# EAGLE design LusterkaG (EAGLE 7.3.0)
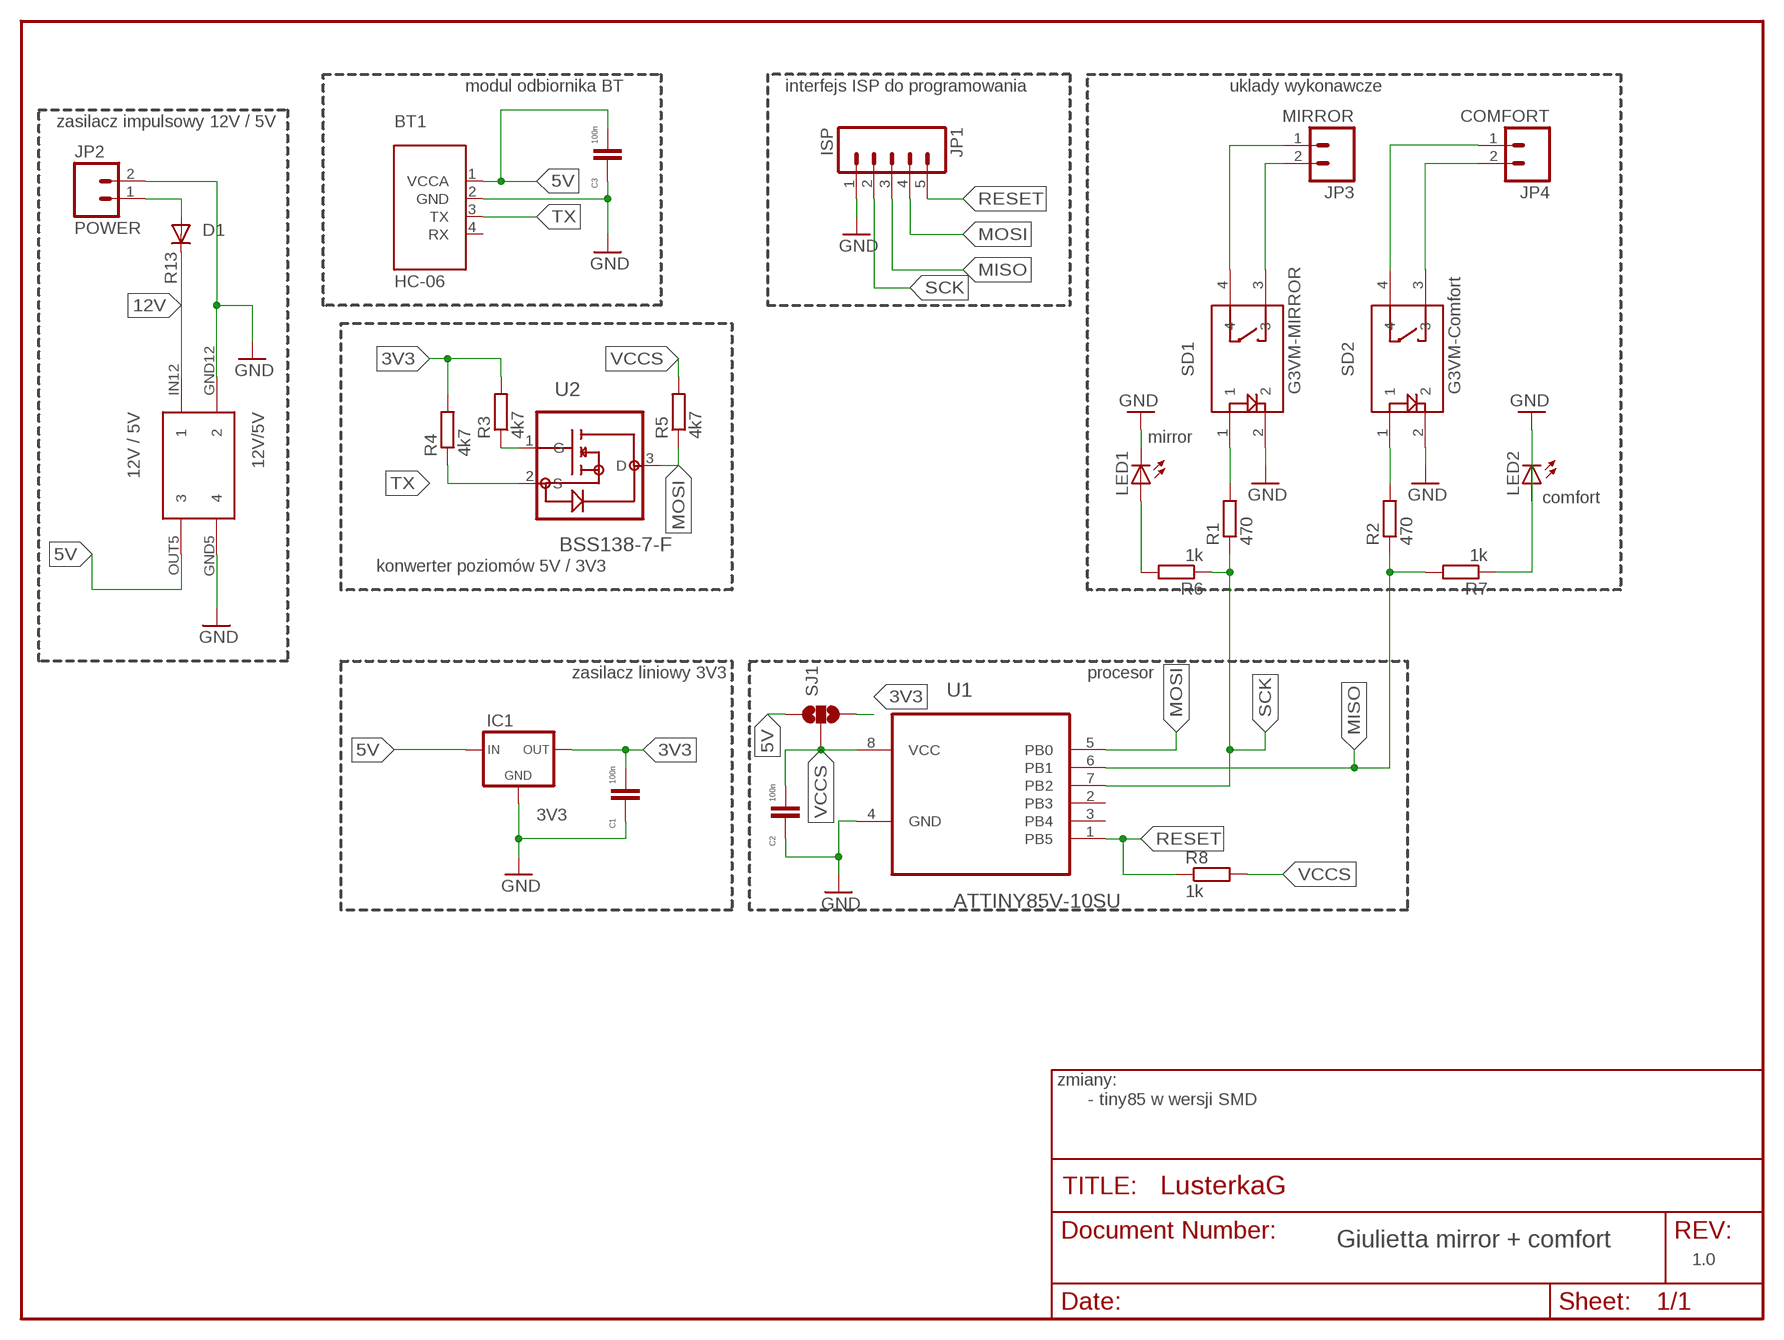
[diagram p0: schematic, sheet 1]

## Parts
12V/5V  12V / 5V  SWITCHING-POWER12V  [SWITCHING-POWER12V]
BT1  HC-06  HC-06-ADAPTER  [HC-06-ADAPETR-HORIZONTAL-V1]
C1  100n  C-EUC0805  [C0805]
C2  100n  C-EUC0805  [C0805]
C3  100n  C-EUC0805  [C0805]
D1  R13  ES2D  [SMB]
IC1  3V3  LM1117TO252  [TO252]
JP1  ISP  M05PTH  [1X05]
JP2  POWER  M02PTH  [1X02]
JP3  MIRROR  M02PTH  [1X02]
JP4  COMFORT  M02PTH  [1X02]
LED1  mirror  LEDCHIP-LED0603  [CHIP-LED0603]
LED2  comfort  LEDCHIP-LED0603  [CHIP-LED0603]
R1  470  R-EU_M0805  [M0805]
R2  470  R-EU_M0805  [M0805]
R3  4k7  R-EU_M0805  [M0805]
R4  4k7  R-EU_M0805  [M0805]
R5  4k7  R-EU_M0805  [M0805]
R6  1k  R-EU_M0805  [M0805]
R7  1k  R-EU_M0805  [M0805]
R8  1k  R-EU_M0805  [M0805]
SD1  G3VM-MIRROR  G3VM-SOLIDRELAY  [G3VM-SOLIDRELAY]
SD2  G3VM-Comfort  G3VM-SOLIDRELAY  [G3VM-SOLIDRELAY]
SJ1  SOLDERJUMPER_2WAYS  [SJ_3]
U1  ATTINY85V-10SU  [SOIC127P798X216-8N]
U2  BSS138-7-F  [SOT95P240X110-3N]

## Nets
3V3: C1.1 IC1.3(OUT) R3.2 R4.2 SJ1.3
5V: 12V/5V.OUT5 BT1.1(VCCA) C3.1 IC1.2(IN) SJ1.1
12V: D1.A JP2.1
GND: 12V/5V.GND5 12V/5V.GND12 BT1.2(GND) C1.2 C2.2 C3.2 IC1.1(GND) JP1.1 JP2.2 LED1.C LED2.A SD1.2 SD2.2 U1.4(GND)
MISO: JP1.3 R2.1 R7.2 U1.6(PB1)
MOSI: JP1.4 R5.1 U1.5(PB0) U2.3(D)
N$1: R1.2 SD1.1
N$2: R2.2 SD2.1
N$3: JP3.1 SD1.4
N$4: JP3.2 SD1.3
N$5: JP4.1 SD2.4
N$6: JP4.2 SD2.3
N$7: R3.1 U2.1(G)
N$8: LED1.A R6.2
N$9: LED2.C R7.1
N$10: 12V/5V.IN12 D1.C
RESET: JP1.5 R8.1 U1.1(PB5)
SCK: JP1.2 R1.1 R6.1 U1.7(PB2)
TX: BT1.3(TX) R4.1 U2.2(S)
VCCS: C2.1 R5.2 R8.2 SJ1.2 U1.8(VCC)
Unconnected: BT1.4(RX) U1.2(PB3) U1.3(PB4)

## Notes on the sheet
- modul odbiornika BT | interfejs ISP do programowania | uklady wykonawcze
- zasilacz impulsowy 12V / 5V
- konwerter poziomów 5V / 3V3
- zasilacz liniowy 3V3 | procesor
- zmiany:
- - tiny85 w wersji SMD
- Giulietta mirror + comfort
- 1.0

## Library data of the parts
12V/5V = switching_power_12V:SWITCHING-POWER12V: switching power from 12 V to +5V
BT1 = HC-05:HC-06-ADAPTER: HC06 4 pin horizontal 14x 100mil - 6x 100 mil
C1-C3 = lcd_C65-lbr:C-EU: CAPACITOR, European symbol
D1 = lcd_C65-lbr:ES2D: DIODE
IC1 = lcd_C65-lbr:LM1117
JP1 = SparkFun-Connectors:M05: Header 5 Standard 5-pin 0.1" header. Use with straight break away headers (SKU : PRT-00116), right angle break away headers (PRT-00553), swiss pins (PRT-00743), machine pins (PRT-00117), and female headers (PRT-00115). Molex polarized connector foot print use with SKU : PRT-08230 with associated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
JP2-JP4 = SparkFun-Connectors:M02: Standard 2-pin 0.1" header. Use with
LED1 LED2 = lcd_C65-lbr:LED: LED
R1-R8 = resistor:R-EU_: RESISTOR, European symbol
SD1 SD2 = G3VM-21GR1:G3VM-SOLIDRELAY: G3VM-21GR by Omron, 250 mA / 20 V
SJ1 = SparkFun-Passives:SOLDERJUMPER_2WAY: Solder Jumper 2 way solder jumper
U1 = Tiny85:ATTINY85V-10SU: 8-bit Microcontroller with In-System Programmable Flash; MPN: ATTINY85V-10SU; OC_FARNELL: 1455166; OC_NEWARK: 58M3799; PACKAGE: SOIC-8; SUPPLIER: Atmel
U2 = BSS138:BSS138-7-F: ENHANCEMENT MODE MOSFET; MPN: BSS138-7-F; OC_FARNELL: 1843693; OC_NEWARK: 12T1442; PACKAGE: SOT-23-3; SUPPLIER: DIODES INC.

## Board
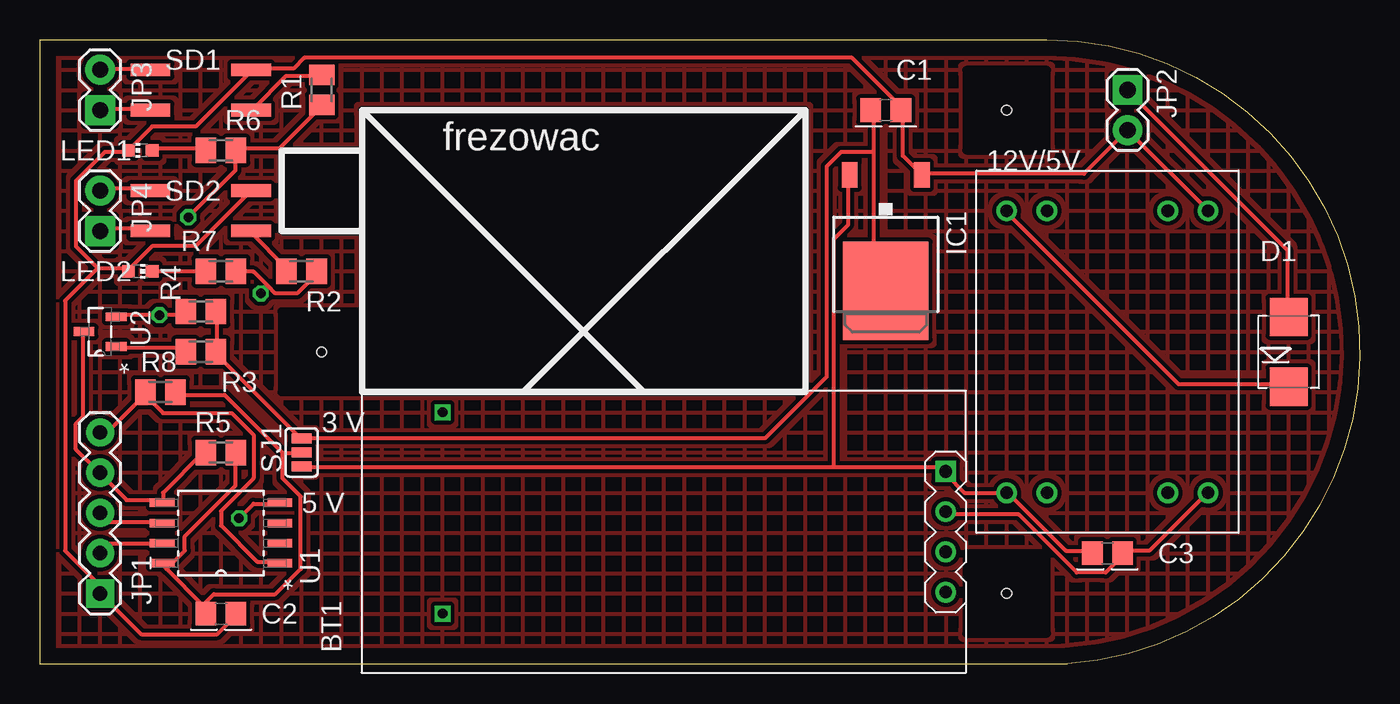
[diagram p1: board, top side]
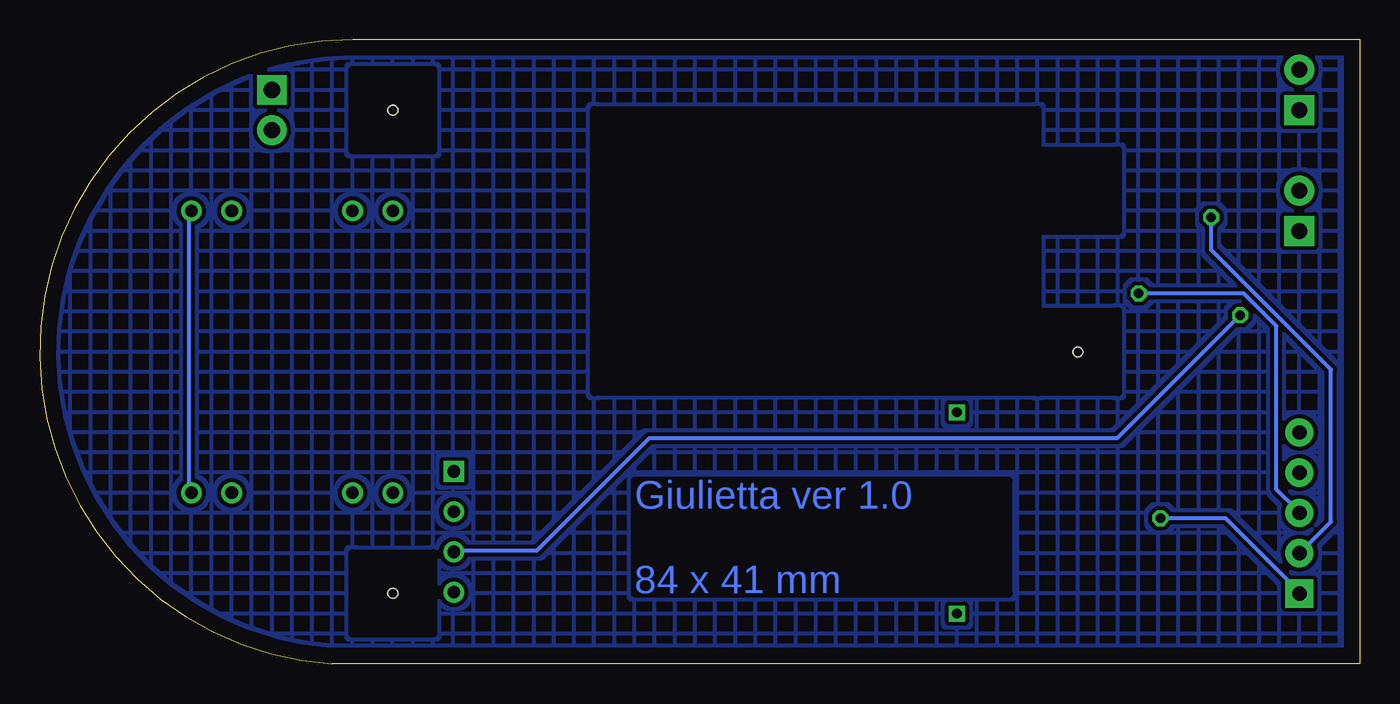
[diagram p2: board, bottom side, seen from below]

Size 83.22 x 39.37 mm. Coordinates in mm from the lower left corner, seen from the top.
Outline: 0,39.37 0,0 64.77,0 arc176 63.5,39.37 0,39.37
Copper layers (1*16): Top 0.035mm / dielectric 1.5mm / Bottom 0.035mm
Design rules "default *": minimum track width 10mil, minimum drill 0.6mm, track to track 8mil, track to pad 0.3mm, pad to pad 0.3mm, via to via 0.5mm, smd to smd 8mil, copper to edge 40mil, drill to drill 8mil, minimum pad ring 10mil, minimum via ring 8mil, stop-mask expansion 4mil, vias tented up to drill 0mil, thermal gap 10mil
Holes 0.6 mm at 60.96,34.93 60.96,4.45 17.78,19.68
tRestrict: area 20.3,17.1 to 48.3,34.9; area 15.2,27.3 to 20.3,32.4; area 15.2,17.1 to 20.3,22.2; area 58.4,32.4 to 63.5,37.5; area 58.4,1.9 to 63.5,7
bRestrict: area 20.3,17.1 to 48.3,34.9; area 15.2,27.3 to 20.3,32.4; area 15.2,17.1 to 20.3,22.2; area 58.4,32.4 to 63.5,37.5; area 58.4,1.9 to 63.5,7

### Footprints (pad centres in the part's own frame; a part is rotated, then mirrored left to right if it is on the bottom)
SWITCHING-POWER12V = drill 0.8: GND5 6.35,-8.89; GND5A 3.81,-8.89; GND12 6.35,8.89; GND12A 3.81,8.89; IN12 -6.35,8.89; IN12A -3.81,8.89; OUT5 -6.35,-8.89; OUT5A -3.81,-8.89
HC-06-ADAPETR-HORIZONTAL-V1 = drill 0.8 square: 1 5.08,0 | drill 0.8: 2 2.54,0; 3 0,0; 4 -2.54,0
C0805 = smd 1.3 x 1.5: 1 -0.95,0; 2 0.95,0
SMB = smd 2.4 x 2.4: A 2.2,0; C -2.2,0
TO252 = smd 1 x 1.6: 1 -2.28,-6.07; 2 2.28,-6.07 | smd 5.4 x 6.2: 3 0,1.23
1X05 = drill 0.9 pad 1.778 square: 1 0,0 | drill 0.9 pad 1.778: 2 2.54,0; 3 5.08,0; 4 7.62,0; 5 10.16,0
1X02 = drill 1.016 pad 1.88 square: 1 0,0 | drill 1.016 pad 1.88: 2 2.54,0
CHIP-LED0603 = smd 0.8 x 0.8: A 0,-0.75; C 0,0.75
M0805 = smd 1.3 x 1.6: 1 -0.95,0; 2 0.95,0
G3VM-SOLIDRELAY = smd 0.8 x 2.5: 1 -1.27,-3.175; 2 1.27,-3.175; 3 1.27,3.175; 4 -1.27,3.175
SJ_3 = smd 0.635 x 1.27: 1 -0.889,0; 2 0,0; 3 0.889,0
SOIC127P798X216-8N = smd 1.549 x 0.533: 1 -3.708,1.905; 2 -3.708,0.635; 3 -3.708,-0.635; 4 -3.708,-1.905; 5 3.708,-1.905; 6 3.708,-0.635; 7 3.708,0.635; 8 3.708,1.905
SOT95P240X110-3N = smd 1.321 x 0.559: 1 -1.016,0.94; 2 -1.016,-0.94; 3 1.016,0

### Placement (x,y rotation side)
12V/5V  67.31,19.68 0 top
BT1  57.12,7.07 90 top
C1  53.34,34.93 0 top
C2  11.43,3.17 0 top
C3  67.31,6.99 0 top
D1  78.74,19.68 90 top
IC1  53.34,24.76 180 top
JP1  3.81,4.45 90 top
JP2  68.58,36.2 270 top
JP3  3.81,34.93 90 top
JP4  3.81,27.3 90 top
LED1  6.35,32.39 90 top
LED2  6.35,24.76 270 top
R1  17.78,36.2 90 top
R2  16.51,24.76 180 top
R3  10.16,19.68 0 top
R4  10.16,22.22 0 top
R5  11.43,13.34 0 top
R6  11.43,32.39 180 top
R7  11.43,24.76 0 top
R8  7.62,17.14 0 top
SD1  10.16,36.2 90 top
SD2  10.16,28.57 90 top
SJ1  16.51,13.34 90 top
U1  11.43,8.26 180 top
U2  3.81,20.95 180 top

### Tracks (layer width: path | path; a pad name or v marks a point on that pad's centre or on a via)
3V3
  Top 0.254: R4.2 11.2,22.22 11.2,19.71 R3.2 11.2,19.48 16.46,14.22 SJ1.3 45.72,14.22 49.61,18.11 49.61,31.37 50.52,32.28 52.58,32.28 | 52.58,32.28 52.58,24.28 53.26,23.6 IC1.3 | 52.58,32.28 52.58,34.8 C1.1
5V
  Top 0.254: C3.1 66.29,7.14 64.69,7.14 61.04,10.79 12V/5V.OUT5 58.29,10.79 57.15,11.94 BT1.1 56.92,12.17 56.69,12.39 50.06,12.39 | 50.06,12.39 16.69,12.39 SJ1.1 | 50.06,12.39 50.06,26.8 50.98,27.71 50.98,30.68 IC1.2
12V
  Top 0.254: D1.A 78.64,22 78.64,26.11 68.58,36.17 JP2.1
GND  (via drill 0.6)
  Top 0.254: C2.2 12.34,3.02 11.2,1.88 6.4,1.88 3.89,4.39 JP1.1 3.66,4.62 3.66,5.08 1.6,7.14 1.6,22.91 3.66,24.97 | v12.57,9.2 13.49,10.11 15.09,10.11 U1.4 | SD2.2 9.83,26.34 7.09,26.34 5.71,24.97 LED2.A 5.49,24.97 3.66,24.97 | 3.66,24.97 2.29,26.34 2.29,30.45 4.12,32.28 5.49,32.28 LED1.C 5.71,32.51 7.09,33.88 9.83,33.88 13.26,37.31 SD1.2 13.49,37.54 16,37.54 16.69,38.23 51.21,38.23 54.41,35.03 C1.2 54.41,34.8 54.41,32.05 55.55,30.91 IC1.1 55.78,30.91 65.84,30.91 JP2.2 12V/5V.GND12 | 12V/5V.GND5 73.61,10.79 69.95,7.14 68.35,7.14 C3.2 68.35,6.91 67.21,5.77 65.38,5.77 61.72,9.42 57.15,9.42 BT1.2
  Bottom 0.254: v12.57,9.2 8.46,9.2 3.89,4.62 JP1.1 | 12V/5V.GND5 73.84,10.79 73.84,28.4 12V/5V.GND12
MISO  (via drill 0.6)
  Top 0.254: 14.4,23.82 14.86,23.37 16.23,23.37 17.6,24.74 R2.1 | 14.4,23.82 13.49,24.74 12.57,24.74 R7.2 | U1.6 7.54,8.97 4.34,8.97 3.89,9.42 JP1.3 | v13.95,23.37 14.4,23.82
  Bottom 0.254: v13.95,23.37 7.32,23.37 5.26,21.31 5.26,11.02 3.89,9.65 JP1.3
MOSI
  Top 0.254: R5.1 10.29,13.31 7.77,10.79 7.77,10.34 U1.5 7.54,10.34 5.49,10.34 3.89,11.94 JP1.4 3.66,12.17 2.29,13.54 2.29,15.14 2.74,15.6 2.74,20.85 U2.3
N$1
  Top 0.254: R1.2 17.6,37.08 15.54,37.08 13.49,35.03 SD1.1
N$2
  Top 0.254: R2.2 15.54,24.97 13.26,27.25 SD2.1
N$3
  Top 0.254: SD1.4 6.86,35.03 3.89,35.03 JP3.1
N$4
  Top 0.254: SD1.3 6.86,37.54 3.89,37.54 JP3.2
N$5
  Top 0.254: SD2.4 6.86,27.48 3.89,27.48 JP4.1
N$6
  Top 0.254: SD2.3 6.86,30 3.89,30 JP4.2
N$7
  Top 0.254: U2.1 5.03,19.94 8.91,19.94 9.14,19.71 R3.1
N$8
  Top 0.254: LED1.A 7.32,32.51 10.29,32.51 R6.2
N$9
  Top 0.254: LED2.C 7.32,24.74 10.29,24.74 R7.1
N$10
  Top 0.254: D1.C 78.64,17.65 71.78,17.65 61.04,28.4 12V/5V.IN12
N$11  (via drill 0.6)
  other vias: 25.4,15.88
N$12  (via drill 0.6)
  other vias: 25.4,3.17
N$13
  pour Top (isolate 0.254, hatched): 0,40.01 63.5,40.01 arc-90 83.82,19.68 arc-82 66.04,-0.64 0,-0.64
N$14
  pour Bottom (isolate 0.254, hatched): 0,40.01 63.5,40.01 arc-90 83.82,19.68 arc-82 66.04,-0.64 0,-0.64
RESET
  Top 0.254: 6.63,16.97 7.77,15.82 12.12,15.82 13.49,14.45 13.49,11.71 11.43,9.65 11.43,8.74 13.72,6.45 15.09,6.45 U1.1 | 6.63,16.97 4.34,14.68 3.89,14.68 JP1.5 | 6.63,16.97 R8.1
SCK  (via drill 0.6)
  Top 0.254: R1.1 17.6,35.03 15.09,32.51 12.57,32.51 R6.1 12.34,32.28 12.34,31.14 v9.37,28.17 | U1.7 7.54,7.6 4.34,7.6 3.89,7.14 JP1.2
  Bottom 0.254: v9.37,28.17 9.37,26.11 1.83,18.57 1.83,8.97 JP1.2
TX  (via drill 0.6)
  Top 0.254: U2.2 5.03,22 v7.54,22 8.91,22 9.14,22.22 R4.1
  Bottom 0.254: v7.54,22 15.32,14.22 44.81,14.22 51.89,7.14 56.92,7.14 BT1.3
VCCS
  Top 0.254: 15.32,13.31 16.46,13.31 SJ1.2 | 15.32,13.31 11.66,16.97 8.69,16.97 R8.2 | 10.29,3.71 10.29,3.25 C2.1 10.29,3.71 | 8,5.99 7.77,6.22 U1.8 | 8,5.99 10.29,3.71 | 8,5.99 9.14,7.14 9.14,8.05 12.34,11.25 12.34,13.31 R5.2 | 15.32,13.31 15.32,11.71 16.46,10.57 16.46,5.99 14.86,4.39 10.97,4.39 10.29,3.71

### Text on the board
Bottom: Giulietta ver 1.0 / / 84 x 41 mm
tPlace: frezowac | 3 V | 5 V
Document: hold for HC-06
